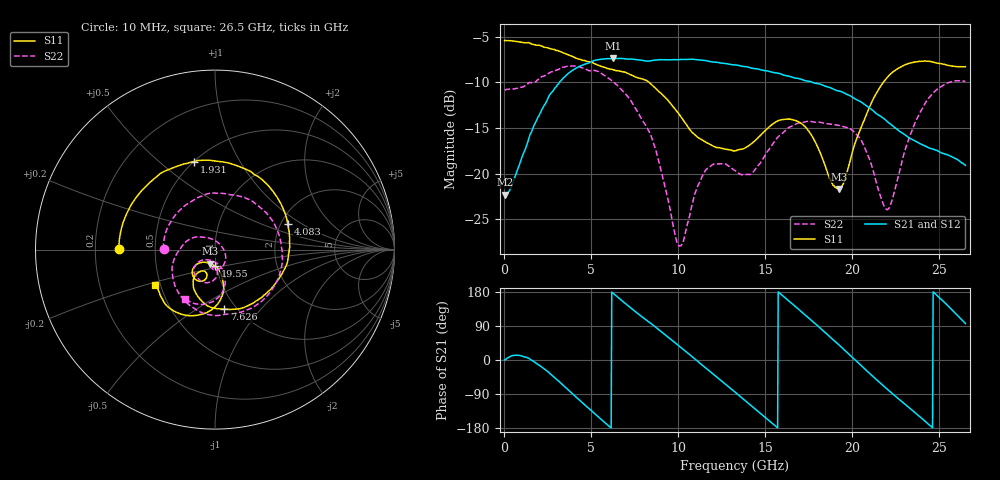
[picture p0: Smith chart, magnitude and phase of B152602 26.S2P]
!  2-Port S-parameters saved by WinCal
! VAR MeasName=S-Parameters (CALIBRATED_DATA) read from VNA (N5242A)
! VAR MeasDate=2016-1-5 16:28:55
! VAR NAME=B152602 26
! VAR FILENAME=B152602 26.S2P
! VAR DATE=2016-1-5 16:28:55
! VAR PHYS_PORTS=1,2
# Hz S DB R 50
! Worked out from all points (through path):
!   801 points, 10 MHz to 26.5 GHz, reference 50 ohm
!   highest |S21| = -7.37 dB at 6.235 GHz (marker M1); lowest = -22.3 dB at 43.11 MHz (marker M2)
!   lowest |S11| = -21.7 dB at 19.22 GHz (marker M3), VSWR 1.18, Z = 47 - j7.43 ohm
!   |S11| at or under -10 dB: 8.318 GHz to 21.78 GHz (13.46 GHz wide, 89.5 % of centre)
!   |S22| runs from -27.9 to -8.2 dB; largest |S21 - S12| = 0.0029
!   S11 on the Smith chart (normalised r, x): 10 MHz: 0.30, +0.00; 1.931 GHz: 0.50, +0.66; 4.083 GHz: 2.17, +0.77; 7.626 GHz: 0.88, -0.66; 19.55 GHz: 0.98, -0.18; 26.5 GHz: 0.47, -0.22
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1e7  -5.44 179.5  -22.27 0.1  -22.28 -0.1  -10.86 179.4
4.31125e7  -5.42 178.3  -22.30 0.9  -22.31 1.0  -10.85 177.7
1.135825e9  -5.66 135.0  -17.61 8.3  -17.61 8.3  -10.43 112.8
1.930525e9  -5.94 103.4  -13.80 -11.9  -13.81 -11.9  -9.72 66.1
3.023238e9  -6.51 60.0  -10.33 -52.1  -10.34 -52.1  -8.64 4.6
4.082838e9  -7.32 19.6  -8.47 -96.3  -8.47 -96.3  -8.22 -47.4
4.447075e9  -7.57 7.2  -8.15 -111.7  -8.14 -111.6  -8.40 -63.2
6.23515e9  -8.61 -47.0  -7.37 176.5  -7.38 176.6  -9.89 -127.7
7.625875e9  -9.47 -81.1  -7.53 124.1  -7.50 124.2  -13.14 -171.7
8.851038e9  -10.96 -108.3  -7.53 80.8  -7.49 80.6  -18.49 143.4
1.00762e10  -13.59 -125.6  -7.51 35.8  -7.48 35.7  -27.89 46.5
1.153315e10  -16.50 -124.4  -7.61 -19.7  -7.61 -19.8  -19.71 -65.3
1.3255e10  -17.49 -114.9  -8.10 -84.7  -8.08 -84.8  -19.66 -98.5
1.421526e10  -16.70 -107.8  -8.45 -121.6  -8.40 -121.6  -19.96 -90.0
1.550665e10  -14.44 -111.7  -8.95 -171.3  -8.90 -171.5  -16.53 -86.6
1.769208e10  -15.90 -139.3  -9.99 102.6  -9.97 102.7  -14.30 -111.5
1.921525e10  -21.67 -107.8  -10.95 40.6  -10.94 40.4  -14.71 -124.4
1.954638e10  -20.77 -89.8  -11.17 26.2  -11.15 26.3  -14.88 -127.0
2.053975e10  -14.78 -75.9  -12.21 -16.1  -12.18 -16.1  -16.44 -139.8
2.209604e10  -9.28 -95.0  -14.45 -80.5  -14.37 -80.7  -23.83 -99.7
2.418212e10  -7.67 -127.9  -16.98 -161.6  -16.94 -162.1  -12.30 -80.5
2.65e10  -8.29 -149.5  -19.09 96.1  -19.08 95.7  -9.89 -121.3
